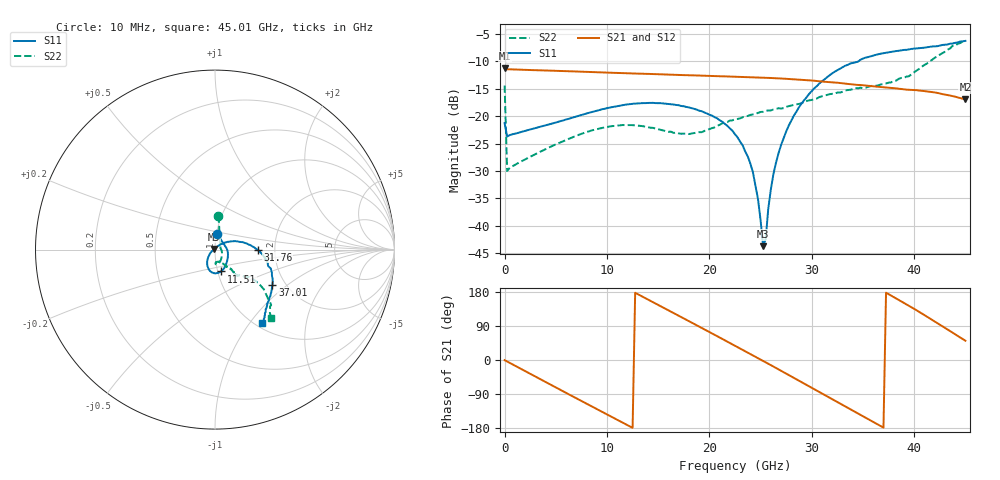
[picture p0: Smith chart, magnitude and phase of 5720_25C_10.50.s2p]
! Device:  ADRF5720
! Description: 0.5dB LSB GaAs MMIC 6-bit Digital Attenuator
! Frequency:  0.000009 -  40 GHz
! Ports:
!	RF1	= Port 1
!	RF2	= Port 2
! Vdd:  3.3 Volt
! Vss:  -3.3 Volt
! Control:  0/3.3 Volt
! State:  10.50 dB attenuation
! Data:  The device was measured using G-S-G Probes on a matrix board.
!  Data was collected using an calibrated 4 port network analyzer.
!  The reference plane for this measurement is at the launchers.
! Note:  Analog Devices supplies this data as a sample of measured data
!  for this product.  Your particular data for this product may vary.
!  Data was taken at 25 degrees C.
!  Analog Devices reserves the right to change this data at anytime.
# GHZ S DB R 45.0
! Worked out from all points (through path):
!   181 points, 10 MHz to 45.01 GHz, reference 45 ohm
!   highest |S21| = -11.23 dB at 10 MHz (marker M1); lowest = -16.9 dB at 45.01 GHz (marker M2)
!   group delay of S21, straight-line fit = 40.8 ps
!   lowest |S11| = -43.8 dB at 25.26 GHz (marker M3), VSWR 1.01, Z = 44.5 + j0.277 ohm
!   |S11| at or under -10 dB: start of sweep to 34.54 GHz
!   |S22| runs from -30.0 to -6.2 dB; largest |S21 - S12| = 0.00041
!   S11 on the Smith chart (normalised r, x): 10 MHz: 1.01, +0.17; 11.51 GHz: 1.04, -0.26; 31.76 GHz: 1.62, -0.00; 37.01 GHz: 1.71, -0.79; 45.01 GHz: 1.08, -1.16
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0.01  -21.25 80.9  -11.23 -0.4  -11.23 -0.4  -14.40 84.2
0.26  -23.71 5.7  -11.42 -4.0  -11.42 -4.0  -30.02 13.2
4.26  -21.54 -31.8  -11.66 -61.8  -11.67 -61.8  -25.79 -41.9
7.76  -19.63 -54.1  -11.88 -111.7  -11.88 -111.6  -23.05 -64.8
11.51  -17.98 -74.5  -12.13 -164.9  -12.13 -164.9  -21.62 -81.5
15.26  -17.62 -92.6  -12.34 141.7  -12.35 141.8  -22.47 -87.9
19.01  -18.99 -109.1  -12.57 88.1  -12.58 88.2  -22.91 -70.2
22.76  -23.87 -129.2  -12.80 34.0  -12.81 34.1  -20.50 -58.6
24.26  -30.24 -144.5  -12.91 12.2  -12.91 12.2  -19.67 -57.3
24.76  -35.19 -153.7  -12.93 4.9  -12.93 5.0  -19.39 -56.9
25.26  -43.75 151.4  -12.97 -2.5  -12.97 -2.4  -19.19 -57.0
25.51  -42.38 85.5  -12.98 -6.2  -12.99 -6.1  -19.02 -57.0
25.76  -36.90 66.5  -13.01 -9.9  -13.01 -9.8  -18.96 -56.3
26.26  -30.61 48.5  -13.04 -17.3  -13.05 -17.2  -18.78 -54.5
27.01  -25.27 37.9  -13.11 -28.4  -13.11 -28.4  -18.60 -54.3
28.26  -19.90 27.0  -13.26 -47.0  -13.26 -47.0  -17.93 -53.3
30.26  -14.90 11.0  -13.53 -77.0  -13.53 -77.0  -16.84 -50.6
31.76  -12.50 -0.1  -13.78 -99.3  -13.78 -99.3  -15.97 -50.3
37.01  -8.49 -31.7  -14.71 -178.4  -14.71 -178.4  -14.13 -46.3
37.76  -8.24 -35.3  -14.83 170.1  -14.84 170.2  -13.82 -44.4
41.76  -7.26 -48.6  -15.59 106.0  -15.59 106.1  -9.70 -38.5
45.01  -6.24 -57.1  -16.94 50.9  -16.94 51.0  -6.16 -50.6
